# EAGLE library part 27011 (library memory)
MEMORY
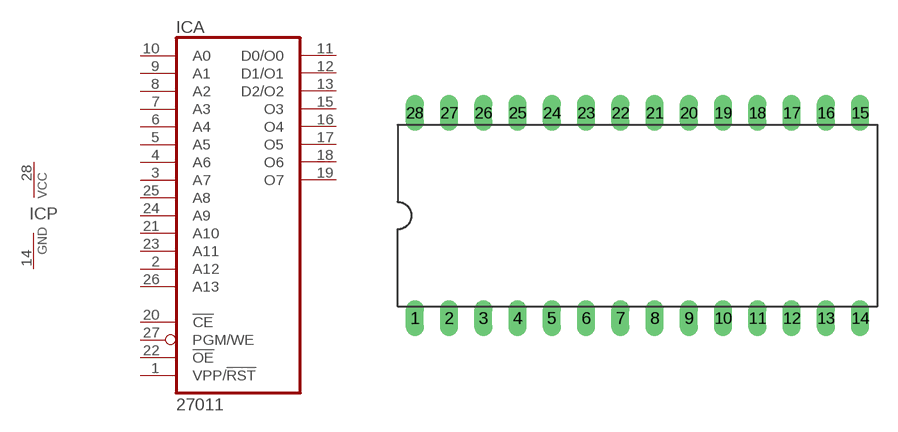
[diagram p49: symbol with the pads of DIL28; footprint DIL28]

Designator prefix IC; gates A=27011 P=PWRN

## 27011  [DIL28]
1  A:VPP/!RST  in
2  A:A12  in
3  A:A7  in
4  A:A6  in
5  A:A5  in
6  A:A4  in
7  A:A3  in
8  A:A2  in
9  A:A1  in
10  A:A0  in
11  A:D0/O0  hiz
12  A:D1/O1  hiz
13  A:D2/O2  hiz
14  P:GND  pwr
15  A:O3  hiz
16  A:O4  hiz
17  A:O5  hiz
18  A:O6  hiz
19  A:O7  hiz
20  A:!CE  in
21  A:A10  in
22  A:!OE  in
23  A:A11  in
24  A:A9  in
25  A:A8  in
26  A:A13  in
27  A:PGM/WE  in
28  P:VCC  pwr

## Footprint DIL28 (pad centres in mm)
Dual In Line Package
drill 0.813 long: 1 -16.51,-7.62; 2 -13.97,-7.62; 3 -11.43,-7.62; 4 -8.89,-7.62; 5 -6.35,-7.62; 6 -3.81,-7.62; 7 -1.27,-7.62; 8 1.27,-7.62; 9 3.81,-7.62; 10 6.35,-7.62; 11 8.89,-7.62; 12 11.43,-7.62; 13 13.97,-7.62; 14 16.51,-7.62; 15 16.51,7.62; 16 13.97,7.62; 17 11.43,7.62; 18 8.89,7.62; 19 6.35,7.62; 20 3.81,7.62; 21 1.27,7.62; 22 -1.27,7.62; 23 -3.81,7.62; 24 -6.35,7.62; 25 -8.89,7.62; 26 -11.43,7.62; 27 -13.97,7.62; 28 -16.51,7.62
